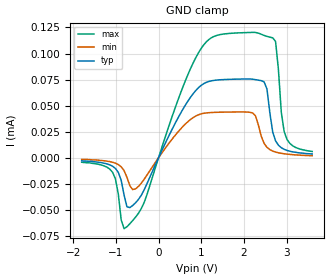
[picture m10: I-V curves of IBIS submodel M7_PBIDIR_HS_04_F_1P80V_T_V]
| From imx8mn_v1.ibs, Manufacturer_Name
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| Submodel
[Submodel]  M7_PBIDIR_HS_04_F_1P80V_T_V
Submodel_type Dynamic_clamp
[GND Clamp]
| Voltage   I(typ)   I(min)   I(max)
-1.8V     -2.916uA   -1.55uA    -4.255uA
-1.076V   -8.106uA   -4.321uA   -13.98uA
-874.1mV  -21.63uA   -8.658uA   -59.66uA
-739.7mV  -46.97uA   -18.72uA   -66.18uA
-470.7mV  -39.97uA   -27.49uA   -53.26uA
931mV     67.06uA    41.19uA    100.4uA
1.867V    75.45uA    43.96uA    119.8uA
2.271V    74.94uA    40.3uA     120.2uA
2.472V    72.84uA    13.86uA    117.4uA
2.741V    16.23uA    5.454uA    111.6uA
2.943V    8.106uA    3.815uA    25.06uA
3.6V      3.631uA    2.027uA    6.043uA
